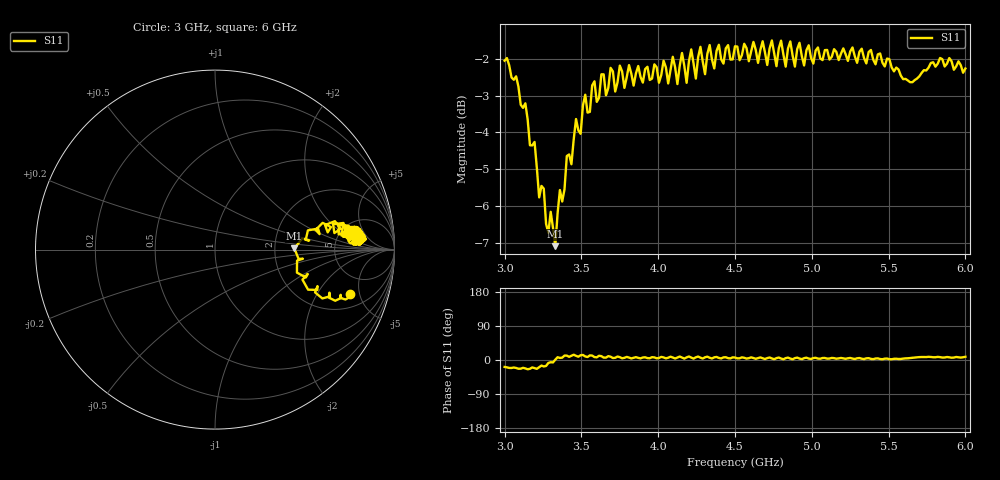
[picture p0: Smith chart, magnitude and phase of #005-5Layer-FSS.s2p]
!  05/08/2025  16:40:39
! Ref Plane: 0.000 mm
# MHZ S MA R  50
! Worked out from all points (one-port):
!   201 points, 3 GHz to 6 GHz, reference 50 ohm
!   lowest |S11| = -7.1 dB at 3.33 GHz (marker M1), VSWR 2.59, Z = 129 + j2.06 ohm
!   |S11| at or under -10 dB: nowhere
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3000  0.7896 -18.4
3150  0.6572 -24.5
3330  0.4424 0.8
3375  0.5086 6.2
3450  0.6179 13.9
3525  0.7099 9.4
3750  0.7776 7.5
4065  0.7354 6.0
4095  0.7992 6.6
4125  0.734 6.5
4155  0.8088 6.5
4185  0.7369 6.9
4215  0.8179 6.4
4245  0.7467 7.1
4275  0.8245 6.1
4305  0.757 7.2
4335  0.8291 5.9
4365  0.7707 7.1
4500  0.826 6.5
4755  0.8078 2.1
4785  0.8206 6.5
4815  0.8052 1.9
4845  0.8206 6.4
4875  0.8026 2.0
4905  0.819 6.3
5250  0.8126 5.4
5625  0.7424 4.5
6000  0.7705 8.6
